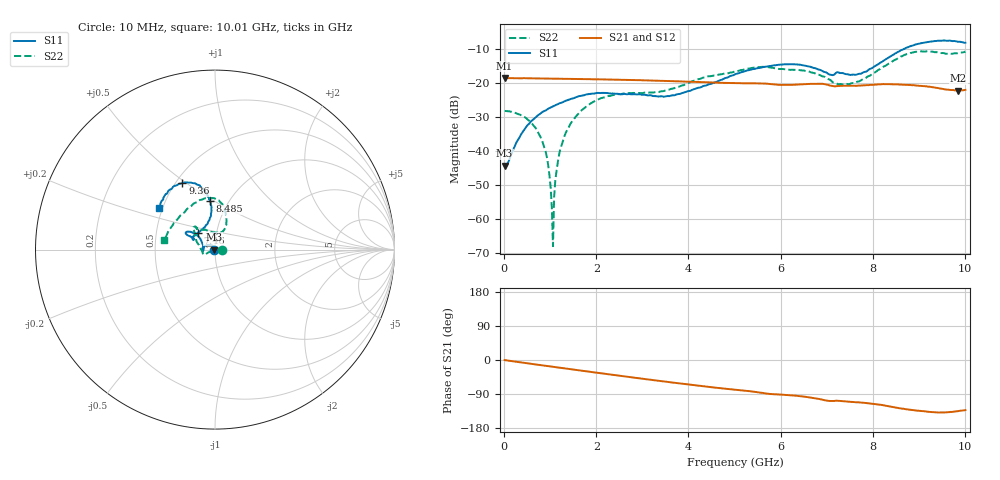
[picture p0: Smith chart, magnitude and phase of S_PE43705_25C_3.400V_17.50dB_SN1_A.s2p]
! Device ID: PE43705
! Serial: 1
! Insertion: A
! Impedance: 50 ohm
! Temp: 25C
! VDD: 3.400V
! Attenuation Step: 17.50dB
#  Hz  S  RI  R  50
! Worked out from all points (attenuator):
!   401 points, 10 MHz to 10.01 GHz, reference 50 ohm
!   highest |S21| = -18.55 dB at 10 MHz (marker M1); lowest = -22.2 dB at 9.86 GHz (marker M2)
!   lowest |S11| = -44.3 dB at 10 MHz (marker M3), VSWR 1.01, Z = 49.4 + j0.0436 ohm
!   |S11| at or under -10 dB: start of sweep to 8.677 GHz
!   |S22| runs from -67.9 to -10.7 dB; largest |S21 - S12| = 0.0013
!   S11 on the Smith chart (normalised r, x): 10 MHz: 0.99, +0.00; 7.46 GHz: 0.81, +0.16; 8.485 GHz: 0.82, +0.48; 9.36 GHz: 0.54, +0.48; 10.01 GHz: 0.48, +0.26
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1e7  -0.00609 0.000441  0.1181 -0.000493  0.1182 -0.000464  0.0389 1.4e-05
4.35e8  -0.0108 0.0175  0.1165 -0.0155  0.1162 -0.0153  0.0315 0.00516
7.35e8  -0.0223 0.0252  0.1138 -0.0254  0.1139 -0.0253  0.0181 0.00551
9.1e8  -0.0299 0.0262  0.1121 -0.0313  0.1121 -0.0311  0.00879 0.00285
9.6e8  -0.0325 0.0267  0.1115 -0.0327  0.1115 -0.0327  0.00556 0.00208
1.01e9  -0.0348 0.0264  0.1108 -0.0343  0.1108 -0.0342  0.00276 0.00091
1.06e9  -0.037 0.0263  0.11 -0.0358  0.1102 -0.0358  -0.000374 0.00015
1.11e9  -0.0393 0.0257  0.1095 -0.0373  0.1095 -0.0372  -0.00345 -0.00135
1.16e9  -0.0415 0.0256  0.109 -0.0387  0.1089 -0.0387  -0.0062 -0.00216
1.26e9  -0.0457 0.0244  0.1075 -0.0419  0.1075 -0.0418  -0.0122 -0.00452
1.685e9  -0.0629 0.0156  0.1006 -0.054  0.1006 -0.054  -0.0366 -0.016
2.26e9  -0.0707 -0.00111  0.0891 -0.0686  0.089 -0.0684  -0.0576 -0.0285
3.36e9  -0.0633 0.00179  0.0617 -0.0883  0.0619 -0.0881  -0.0737 -0.00462
5.01e9  -0.1043 0.0843  0.0199 -0.0975  0.0203 -0.0974  -0.1139 0.0944
6.01e9  -0.158 0.0985  -0.00231 -0.0936  -0.0018 -0.0937  -0.1037 0.1224
6.685e9  -0.1498 0.0783  -0.0167 -0.0956  -0.0165 -0.0956  -0.0837 0.1146
7.46e9  -0.0953 0.0944  -0.0311 -0.0855  -0.0308 -0.0854  0.0147 0.0949
8.36e9  -0.0198 0.2401  -0.0514 -0.0814  -0.0515 -0.0815  0.0624 0.1856
8.485e9  -0.0263 0.2697  -0.0551 -0.0781  -0.055 -0.0784  0.0568 0.2121
9.36e9  -0.182 0.3702  -0.0636 -0.0571  -0.0635 -0.0572  -0.1034 0.2635
9.86e9  -0.2887 0.2787  -0.0546 -0.0549  -0.0546 -0.0548  -0.2462 0.1213
1.001e10  -0.3135 0.2309  -0.0533 -0.0586  -0.0537 -0.0592  -0.2845 0.0537
